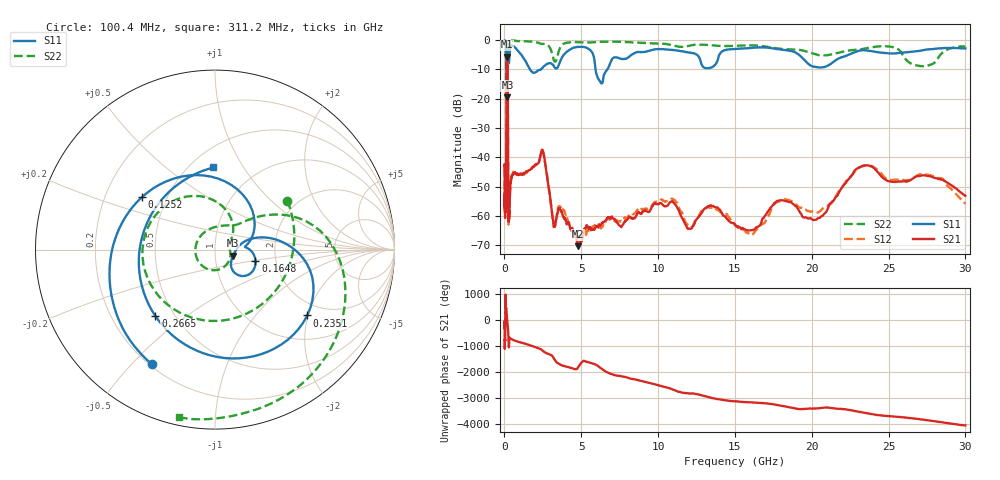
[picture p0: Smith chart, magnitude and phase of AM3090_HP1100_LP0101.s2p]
! Date/Time: Thu, Feb 28, 2019 2:06 PM
! Network Analyzer: Agilent Technologies E8364B Rev: A.07.50.67
! Sweep from 0.010 to 30.000 GHz, 1601 Points, Sweep Type: LOG
! Power Supply: 5.023 V, 0.002 A
# Hz S DB R 50
!freq MagS11 AngS11 MagS21 AngS21 MagS12 AngS12 MagS22 AngS22
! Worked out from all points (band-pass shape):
!   1601 points, 10 MHz to 30 GHz, reference 50 ohm
!   highest |S21| = -5.68 dB at 169 MHz (marker M1); lowest = -70.3 dB at 4.781 GHz (marker M2)
!   |S21| within 3 dB of the highest: 141.3 MHz to 206.5 MHz (65.21 MHz wide, 37.5 % of centre)
!   lowest |S11| = -19.5 dB at 196.4 MHz (marker M3), VSWR 1.24, Z = 60.9 - j4.26 ohm
!   |S11| at or under -10 dB: 136.3 MHz to 216.2 MHz (79.94 MHz wide, 45.3 % of centre); 1.657 GHz to 2.378 GHz (721.6 MHz wide, 35.8 % of centre); 5.925 GHz to 6.698 GHz (772.7 MHz wide, 12.2 % of centre)
!   |S22| runs from -21.9 to -0.1 dB; largest |S21 - S12| = 0.013
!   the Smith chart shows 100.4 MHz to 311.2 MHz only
!   S11 on the Smith chart (normalised r, x): 100.4 MHz: 0.21, -0.57; 125.2 MHz: 0.36, +0.28; 164.8 MHz: 1.56, -0.21; 235.1 MHz: 1.62, -1.98; 266.5 MHz: 0.39, -0.39; 311.2 MHz: 0.64, +0.75
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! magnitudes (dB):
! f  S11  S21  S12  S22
! 10 MHz  -0.3  -43.0  -44.1  -0.6
! 38.04 MHz  -0.4  -56.3  -57.8  -1.3
! 100.4 MHz  -2.7  -54.1  -52.8  -6.3
! 125.2 MHz  -6.0  -25.8  -25.7  -7.8
! 144.7 MHz  -14.7  -7.5  -7.4  -19.3
! 164.8 MHz  -12.6  -5.7  -5.7  -19.4
! 169 MHz  -12.3  -5.7  -5.7  -18.9
! 196.4 MHz  -19.5  -6.8  -6.8  -18.0
! 215.9 MHz  -10.1  -13.7  -13.6  -10.9
! 235.1 MHz  -4.0  -39.9  -39.0  -2.6
! 266.5 MHz  -6.1  -61.3  -62.0  -0.8
! 311.2 MHz  -6.8  -58.9  -60.9  -0.4
! 550.5 MHz  -2.0  -45.8  -45.6  -0.2
! 2.084 GHz  -10.8  -42.4  -42.3  -0.8
! 2.507 GHz  -9.3  -38.0  -37.9  -1.3
! 3.188 GHz  -8.6  -62.3  -63.1  -6.4
! 4.781 GHz  -2.3  -70.3  -67.3  -0.7
! 6.234 GHz  -14.2  -63.3  -63.9  -0.6
! 7.926 GHz  -6.3  -61.5  -60.8  -0.7
! 15.97 GHz  -2.7  -64.9  -66.5  -1.8
! 23.59 GHz  -3.6  -42.7  -42.8  -2.8
! 30 GHz  -2.9  -53.1  -55.8  -2.2
